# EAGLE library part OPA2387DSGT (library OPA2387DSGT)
Precision Amplifiers Ultra-high precision, zero-drift, low-input-bias-current op amp Source: Datasheet
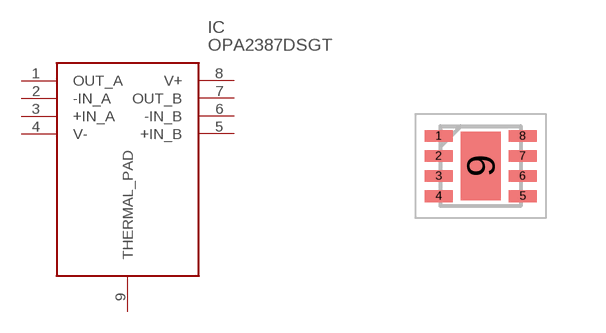
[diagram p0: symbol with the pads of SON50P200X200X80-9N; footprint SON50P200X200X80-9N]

Designator prefix IC

## OPA2387DSGT (Description: Precision Amplifiers Ultra-high precision, zero-drift, low-input-bias-current op amp; Height: 0.8mm; Manufacturer_Name: Texas Instruments; Manufacturer_Part_Number: OPA2387DSGT; Mouser_Part_Number: 595-OPA2387DSGT; Mouser_Price-Stock: https://www.mouser.co.uk/ProductDetail/Texas-Instruments/OPA2387DSGT?qs=MyNHzdoqoQIl7LJ1IzdkFA%3D%3D)  [SON50P200X200X80-9N]
1  OUT_A
2  -IN_A
3  +IN_A
4  V-
5  +IN_B
6  -IN_B
7  OUT_B
8  V+
9  THERMAL_PAD

## Footprint SON50P200X200X80-9N (pad centres in mm)
WSON DSG0008A
smd 0.7 x 0.3: 1 -1.05,0.75; 2 -1.05,0.25; 3 -1.05,-0.25; 4 -1.05,-0.75; 5 1.05,-0.75; 6 1.05,-0.25; 7 1.05,0.25; 8 1.05,0.75
smd 1 x 1.7: 9 0,0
